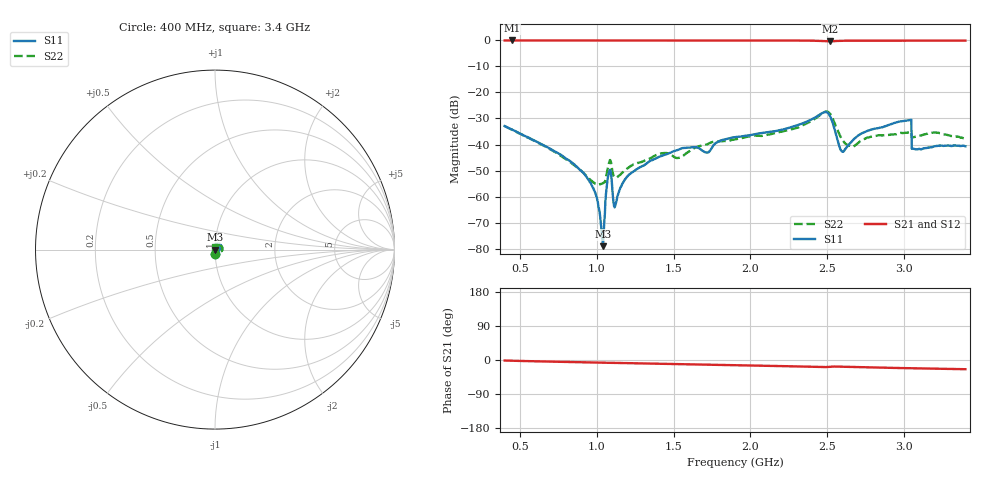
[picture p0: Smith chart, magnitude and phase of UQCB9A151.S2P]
!  Part Number  UQCB9A151	Mounting Orientation: Vertical
!  Description: RF capacitors
!  Application: Coupling, Bypass, Tuning, DC Block
!  Filters, Matching
# GHZ S DB R 50
! Freq  |S11|  S11 Ph  |S21|  S21 Ph  |S12|  S12 Ph  |S22|  S22 Ph
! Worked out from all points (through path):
!   801 points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, 400 MHz to 3.4 GHz, reference 50 ohm
!   highest |S21| = -0.01 dB at 449 MHz (marker M1); lowest = -0.4 dB at 2.519 GHz (marker M2)
!   group delay of S21, straight-line fit = 20.6 ps
!   lowest |S11| = -79.1 dB at 1.041 GHz (marker M3), VSWR 1.00, Z = 50 + j0.00735 ohm
!   |S11| at or under -10 dB: start of sweep to end of sweep
!   |S22| runs from -55.5 to -27.3 dB; largest |S21 - S12| = 0.0014
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0.4  -32.89 -88.6  -0.01 -1.4  -0.01 -1.4  -32.93 -89.3
0.449  -34.30 -88.6  -0.01 -1.9  -0.01 -1.9  -34.34 -89.4
0.903  -50.40 -82.1  -0.02 -6.0  -0.02 -6.0  -50.30 -65.6
0.989  -58.35 -79.6  -0.02 -6.7  -0.02 -6.7  -55.04 -27.9
1.03  -72.23 -54.0  -0.02 -7.0  -0.02 -7.0  -55.12 4.6
1.041  -79.07 41.3  -0.02 -7.1  -0.03 -7.1  -54.77 13.7
1.071  -53.03 73.3  -0.03 -7.3  -0.03 -7.3  -49.23 38.3
1.079  -50.86 54.1  -0.04 -7.4  -0.04 -7.4  -47.27 29.9
1.124  -62.69 56.2  -0.02 -7.6  -0.02 -7.7  -52.76 13.8
1.206  -51.85 84.7  -0.02 -8.3  -0.02 -8.3  -48.92 44.5
1.401  -44.85 90.4  -0.02 -9.8  -0.02 -9.8  -43.74 52.6
1.533  -41.98 89.2  -0.03 -10.8  -0.03 -10.9  -45.11 56.1
1.72  -43.08 92.9  -0.04 -12.3  -0.04 -12.3  -39.89 67.8
1.9  -37.15 93.1  -0.03 -13.6  -0.04 -13.6  -38.00 62.5
2.403  -30.24 77.0  -0.09 -18.0  -0.10 -18.1  -30.80 48.7
2.519  -29.11 14.1  -0.37 -17.8  -0.37 -17.9  -28.20 -10.7
2.601  -42.82 41.8  -0.13 -17.8  -0.14 -17.9  -38.40 -20.8
2.665  -38.54 81.3  -0.09 -18.5  -0.10 -18.6  -40.90 12.8
2.901  -32.51 84.9  -0.07 -20.6  -0.07 -20.6  -36.31 33.0
3.033  -30.72 83.3  -0.08 -21.6  -0.07 -21.6  -35.30 42.0
3.066  -41.70 21.9  -0.07 -21.8  -0.07 -21.8  -37.15 88.1
3.4  -40.70 40.1  -0.06 -24.3  -0.06 -24.4  -37.71 82.6
